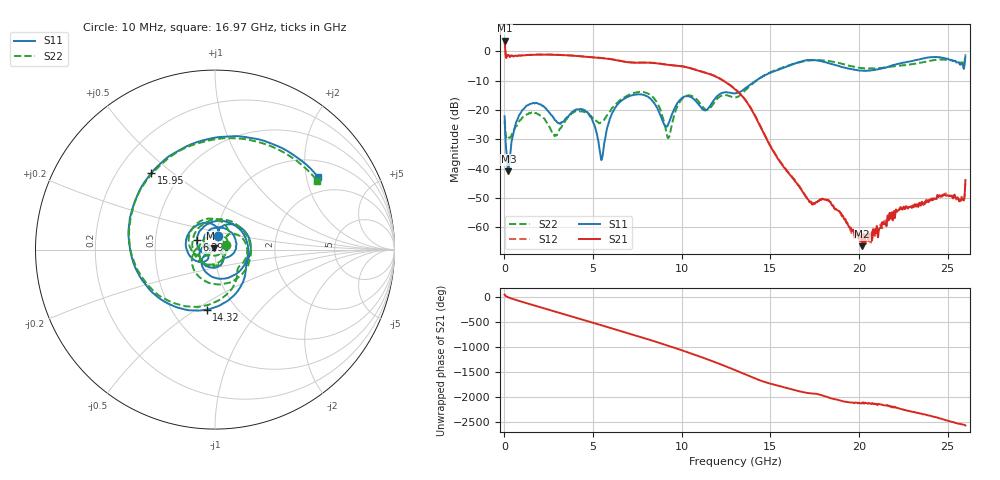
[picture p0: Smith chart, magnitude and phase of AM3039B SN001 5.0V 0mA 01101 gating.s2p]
!Agilent Technologies,E8364B,MY43040894,A.07.50.67
!Agilent E8364B: A.07.50.67
!Date: Tuesday, June 28, 2016 08:06:27
!Correction: S11(Full 2 Port(1,2))
!S21(Full 2 Port(1,2))
!S12(Full 2 Port(1,2))
!S22(Full 2 Port(1,2))
!S2P File: Measurements: S11, S21, S12, S22:
# Hz S  dB  R 50
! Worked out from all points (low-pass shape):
!   1601 points, 10 MHz to 26 GHz, reference 50 ohm
!   highest |S21| = 3.68 dB at 10 MHz (marker M1); lowest = -66.5 dB at 20.18 GHz (marker M2)
!   |S21| within 3 dB of the highest: start of sweep to 44.16 MHz
!   lowest |S11| = -40.9 dB at 221.2 MHz (marker M3), VSWR 1.02, Z = 49.5 + j0.715 ohm
!   |S11| at or under -10 dB: start of sweep to 14.18 GHz
!   |S22| runs from -29.8 to -1.0 dB; largest |S21 - S12| = 0.025
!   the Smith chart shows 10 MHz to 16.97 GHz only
!   S11 on the Smith chart (normalised r, x): 10 MHz: 1.02, +0.16; 6.296 GHz: 0.81, +0.09; 14.32 GHz: 0.74, -0.55; 15.95 GHz: 0.34, +0.42; 16.97 GHz: 1.48, +2.35
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1e7  -22.16 76.9  3.68 40.8  3.75 41.6  -23.80 21.3
2.211688e8  -40.92 126.6  -1.26 -13.9  -1.22 -13.7  -29.37 -62.1
1.634375e9  -17.57 58.4  -1.15 -170.5  -1.10 -170.4  -20.67 63.5
2.657731e9  -21.83 -31.1  -1.13 84.0  -1.06 84.3  -27.21 -30.5
3.486162e9  -22.69 -49.1  -1.32 -1.5  -1.28 -1.3  -23.25 -46.8
4.347081e9  -19.81 -125.5  -1.69 -91.4  -1.66 -91.3  -20.43 -151.3
5.240488e9  -28.86 142.6  -2.15 175.2  -2.11 175.3  -24.03 43.1
6.296331e9  -18.80 152.3  -2.97 61.9  -2.92 62.0  -17.87 171.6
7.660806e9  -14.63 -19.7  -3.84 -79.7  -3.80 -79.8  -13.83 -33.8
8.684162e9  -20.16 -139.4  -4.13 166.0  -4.06 166.1  -18.33 -171.1
1.001615e10  -15.89 177.0  -5.09 12.3  -5.07 12.5  -16.22 161.4
1.146184e10  -19.68 80.5  -7.51 -167.4  -7.42 -167.1  -19.99 48.8
1.3005e10  -14.31 -19.8  -12.87 -20.0  -12.77 -19.6  -15.71 -37.5
1.432074e10  -9.44 -97.8  -24.17 147.3  -24.00 147.3  -9.44 -108.7
1.594512e10  -5.12 129.7  -40.94 -18.7  -40.67 -19.1  -4.99 121.4
1.696848e10  -3.07 35.0  -49.34 -108.6  -49.16 -108.0  -3.27 33.7
1.734208e10  -2.90 -2.7  -52.15 -125.1  -51.66 -124.3  -3.03 0.5
1.839792e10  -4.21 -103.1  -51.51 141.5  -51.46 142.4  -3.38 -92.8
2.018474e10  -6.59 118.2  -66.47 46.1  -64.54 46.8  -5.70 128.5
2.167916e10  -5.12 17.0  -57.69 -9.9  -56.11 -5.9  -5.29 23.5
2.424568e10  -1.92 177.7  -50.13 129.6  -49.84 132.1  -2.95 -166.6
2.6e10  -1.63 -20.7  -44.10 -40.4  -43.56 -41.6  -0.99 10.0
